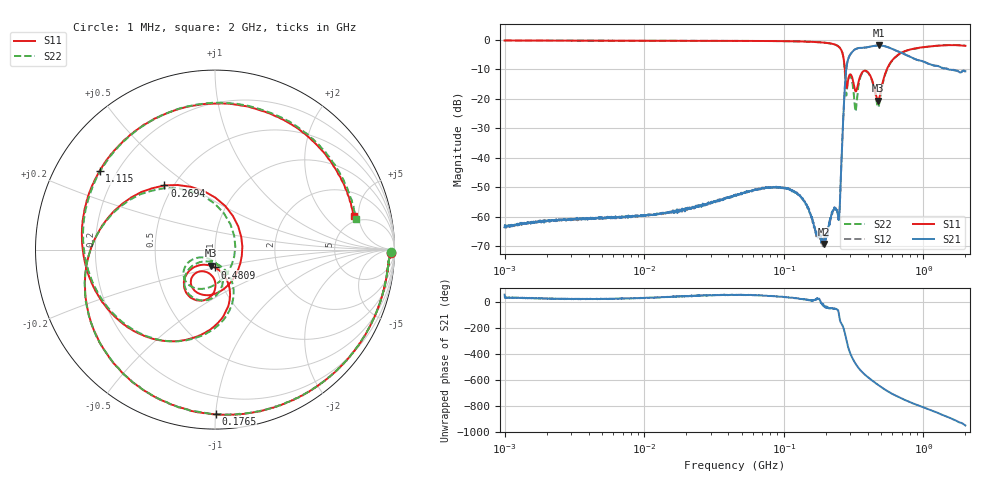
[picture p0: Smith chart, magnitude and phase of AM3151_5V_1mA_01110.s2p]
! Date/Time: Fri Jun 26 10:38:16 2020
! Network Analyzer:  Rev:
! Sweep from 1000000.0 to 2000000000.0, 1601 Points ! Power Supply: 0 V, 0 A
# HZ S DB R 50
!freq MagS11 AngS11 MagS21 AngS21 MagS12 AngS12 MagS22 AngS22
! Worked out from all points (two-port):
!   1601 points, 1 MHz to 2 GHz, reference 50 ohm
!   highest |S21| = -1.86 dB at 480.9 MHz (marker M1); lowest = -69.3 dB at 195 MHz (marker M2)
!   |S21| within 3 dB of the highest: 300.1 MHz to 735.2 MHz (435.1 MHz wide, 84.1 % of centre)
!   lowest |S11| = -20.6 dB at 474.1 MHz (marker M3), VSWR 1.20, Z = 47 - j8.53 ohm
!   |S11| at or under -10 dB: 273.8 MHz to 547.3 MHz (273.5 MHz wide, 66.6 % of centre)
!   |S22| runs from -24.3 to -0.2 dB; largest |S21 - S12| = 0.0071
!   S11 on the Smith chart (normalised r, x): 1 MHz: 59, -49; 176.5 MHz: 0.09, -1.00; 269.4 MHz: 0.45, +0.40; 480.9 MHz: 0.98, -0.20; 1.115 GHz: 0.14, +0.30; 2 GHz: 4.25, +4.32
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1000000  -0.17 -0.9  -63.54 53.3  -63.97 8.6  -0.18 -0.9
3555161  -0.23 -2.0  -60.95 18.8  -60.86 18.9  -0.23 -2.0
1.263916e7  -0.28 -6.2  -59.19 30.9  -59.06 31.7  -0.27 -6.1
4.493426e7  -0.32 -21.2  -52.67 51.5  -52.47 51.7  -0.31 -21.1
1.066767e8  -0.43 -51.1  -50.40 32.6  -50.57 31.8  -0.43 -50.9
1.589914e8  -0.63 -79.2  -60.09 5.8  -60.71 6.6  -0.65 -78.9
1.765073e8  -0.74 -89.7  -66.01 20.9  -65.43 25.5  -0.75 -89.5
1.950242e8  -0.90 -102.2  -69.25 -38.0  -67.85 -40.2  -0.91 -102.2
2.461404e8  -2.20 -157.1  -60.96 -75.4  -60.75 -76.8  -2.16 -156.4
2.544631e8  -2.91 -174.5  -50.68 -154.9  -50.53 -154.6  -2.85 -173.6
2.693907e8  -6.84 128.2  -22.12 148.1  -22.12 148.0  -7.03 129.8
2.811581e8  -16.29 6.3  -9.42 61.4  -9.42 61.5  -18.88 -19.8
2.962411e8  -11.81 -98.0  -5.29 -24.9  -5.29 -24.9  -12.24 -121.5
3.226871e8  -16.75 -123.7  -3.22 -107.3  -3.24 -107.5  -22.48 -144.2
3.721142e8  -10.59 -105.7  -2.62 169.2  -2.61 168.9  -10.79 -101.2
4.74129e8  -20.64 -104.3  -1.89 80.4  -1.88 80.3  -22.88 -102.6
4.809347e8  -20.07 -90.8  -1.86 75.7  -1.88 75.6  -22.04 -84.3
5.652395e8  -8.64 -82.3  -2.55 26.4  -2.55 26.4  -8.77 -78.8
7.340157e8  -3.83 -136.1  -4.85 -34.4  -4.89 -34.5  -3.90 -135.9
1.114967e9  -2.18 145.8  -8.24 -111.2  -8.24 -111.3  -2.20 143.1
1.511136e9  -1.76 83.2  -10.02 -168.2  -9.90 -169.0  -1.72 80.2
2e9  -1.99 13.6  -10.64 129.3  -10.77 128.6  -1.88 12.4
